(* Logix 5000 AddOnInstructionDefinition export AMCI_ANG1E_Jog_CCW; software revision 20.03 *)

ADD_ON_INSTRUCTION AMCI_ANG1E_Jog_CCW   (* revision 5.0, vendor AMCI, ExecuteEnableInFalse *)
// Revision note:
// Version 5.0 added the (hidden) ability to program the motor current and unlatched the error bit if the rung goes false.
VAR_INPUT
   Axis_Status_Bits : DINT; {required}
   slot_axis_number : INT; {required}
   Programmed_Speed : DINT; {required}
   Acceleration : INT; {required}
   Deceleration : INT; {required}
   motor_current : INT;
   jerk : INT;
END_VAR
VAR_IN_OUT
   AMCI_ANG1E_output_data : INT[10]; {required}
END_VAR
VAR_OUTPUT
   EN : BOOL; {access Read Only, visible}
   Jog_CCW_Occurring : BOOL; {access Read Only, visible}
   ER : BOOL; {access Read Only, visible}
END_VAR
VAR
   Upper_Result_X_1000 : DINT;
   command_data_block : INT[10];
        [0]   // Command Bits MSW
        [1]   // Command Bits LSW
        [2]   // Upper Target Position
        [3]   // Lower Target Position
        [4]   // Upper Programmed Speed
        [5]   // Lower Programmed Speed
   index : INT;
END_VAR

ROUTINE EnableInFalse   (* ladder *)
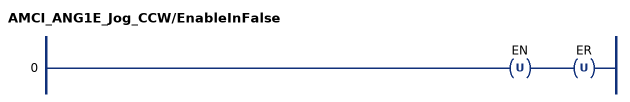
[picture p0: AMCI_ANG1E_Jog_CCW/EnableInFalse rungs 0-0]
   0: OTU(EN)OTU(ER);
END_ROUTINE

ROUTINE Logic   (* ladder *)
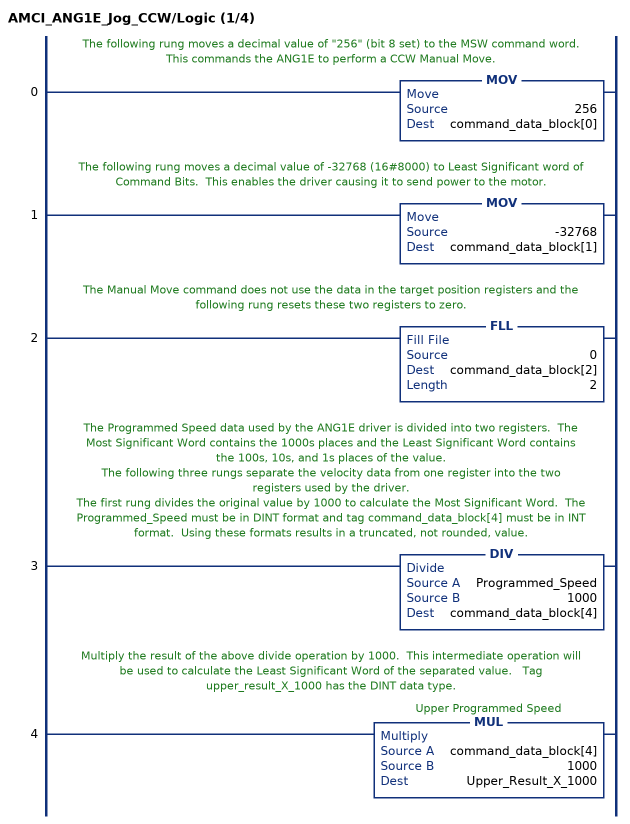
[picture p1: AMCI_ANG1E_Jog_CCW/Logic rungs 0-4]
   // The following rung moves a decimal value of "256" (bit 8 set) to the MSW command word.  This commands the ANG1E to perform a CCW Manual Move.
   0: MOV(256,command_data_block[0]);
   // The following rung moves a decimal value of -32768 (16#8000) to Least Significant word of Command Bits.  This enables the driver causing it to send power to the motor.
   1: MOV(-32768,command_data_block[1]);
   // The Manual Move command does not use the data in the target position registers and the following rung resets these two registers to zero.
   2: FLL(0,command_data_block[2],2);
   // The Programmed Speed data used by the ANG1E driver is divided into two registers.  The Most Significant Word contains the 1000s places and the Least Significant Word contains the 100s, 10s, and 1s places of the value.
   // The following three rungs separate the velocity data from one register into the two registers used by the driver.
   // The first rung divides the original value by 1000 to calculate the Most Significant Word.  The Programmed_Speed must be in DINT format and tag command_data_block[4] must be in INT format.  Using these formats results in a truncated, not rounded, value.
   3: DIV(Programmed_Speed,1000,command_data_block[4]);
   // Multiply the result of the above divide operation by 1000.  This intermediate operation will be used to calculate the Least Significant Word of the separated value.   Tag upper_result_X_1000 has the DINT data type.
   4: MUL(command_data_block[4],1000,Upper_Result_X_1000);
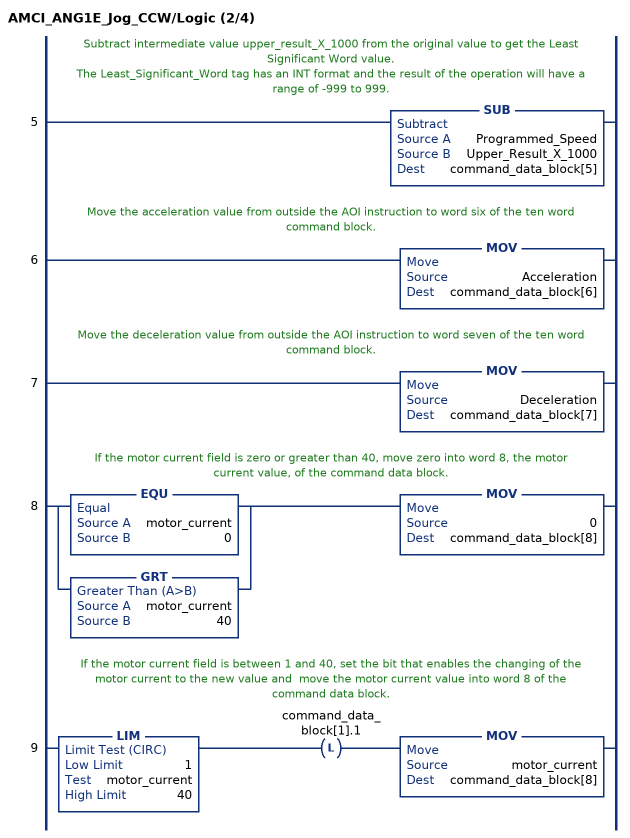
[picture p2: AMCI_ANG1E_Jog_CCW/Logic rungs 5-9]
   // Subtract intermediate value upper_result_X_1000 from the original value to get the Least Significant Word value.
   // The Least_Significant_Word tag has an INT format and the result of the operation will have a range of -999 to 999.
   5: SUB(Programmed_Speed,Upper_Result_X_1000,command_data_block[5]);
   // Move the acceleration value from outside the AOI instruction to word six of the ten word command block.
   6: MOV(Acceleration,command_data_block[6]);
   // Move the deceleration value from outside the AOI instruction to word seven of the ten word command block.
   7: MOV(Deceleration,command_data_block[7]);
   // If the motor current field is zero or greater than 40, move zero into word 8, the motor current value, of the command data block.
   8: [EQU(motor_current,0) ,GRT(motor_current,40) ]MOV(0,command_data_block[8]);
   // If the motor current field is between 1 and 40, set the bit that enables the changing of the motor current to the new value and  move the motor current value into word 8 of the command data block.
   9: LIM(1,motor_current,40)OTL(command_data_block[1].1)MOV(motor_current,command_data_block[8]);
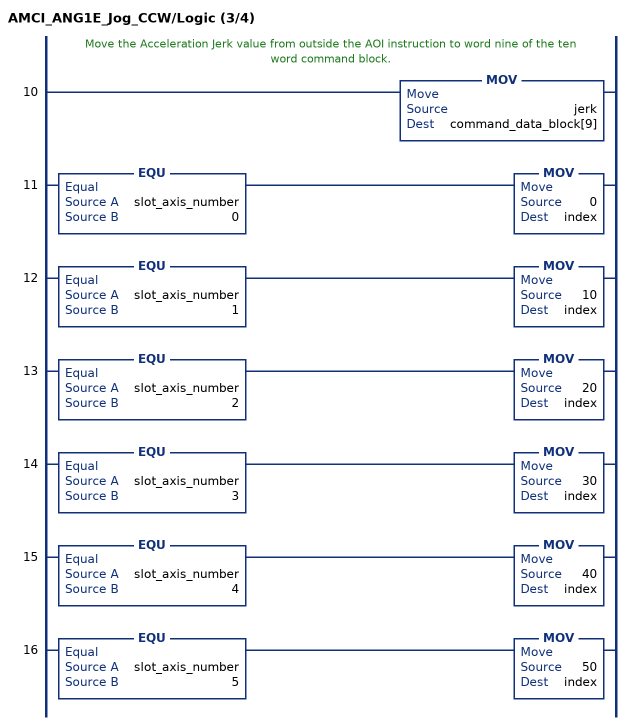
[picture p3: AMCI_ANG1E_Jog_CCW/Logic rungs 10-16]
   // Move the Acceleration Jerk value from outside the AOI instruction to word nine of the ten word command block.
   10: MOV(jerk,command_data_block[9]);
   11: EQU(slot_axis_number,0)MOV(0,index);
   12: EQU(slot_axis_number,1)MOV(10,index);
   13: EQU(slot_axis_number,2)MOV(20,index);
   14: EQU(slot_axis_number,3)MOV(30,index);
   15: EQU(slot_axis_number,4)MOV(40,index);
   16: EQU(slot_axis_number,5)MOV(50,index);
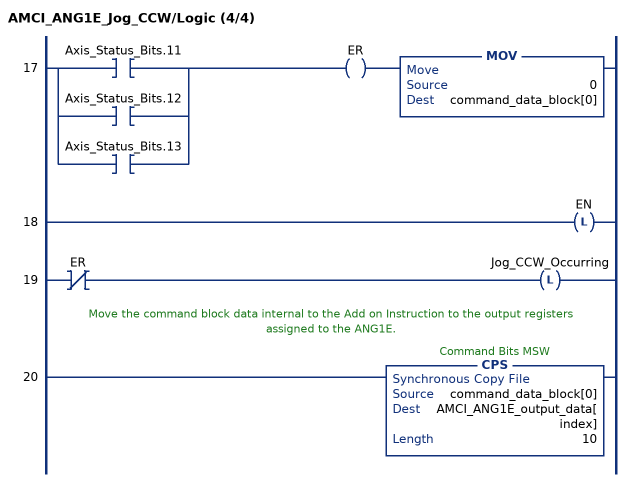
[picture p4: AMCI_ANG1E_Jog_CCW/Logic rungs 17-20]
   17: [XIC(Axis_Status_Bits.11) ,XIC(Axis_Status_Bits.12) ,XIC(Axis_Status_Bits.13) ]OTE(ER)MOV(0,command_data_block[0]);
   18: OTL(EN);
   19: XIO(ER)OTL(Jog_CCW_Occurring);
   // Move the command block data internal to the Add on Instruction to the output registers assigned to the ANG1E.
   20: CPS(command_data_block[0],AMCI_ANG1E_output_data[index],10);
END_ROUTINE
END_ADD_ON_INSTRUCTION
